VAR_GLOBAL CONSTANT
	cOversamples 	: UDINT 	:= 10;		// number of oversamples
	cBufferLength	: UDINT		:= 1600;	// buffer size
	cWindowLength	: UDINT		:= 3200;	// internal buffer size with 50% overlapping
	cFFTResult 		: UDINT 	:= 2049;	// result of mag. spectrum (cFFTLength/2+1)
	cFFTLength		: UDINT		:= 4096;	// length of FFT for mag. spectrum	
END_VAR
